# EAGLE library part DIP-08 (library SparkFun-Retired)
DIP Switch 8 Position
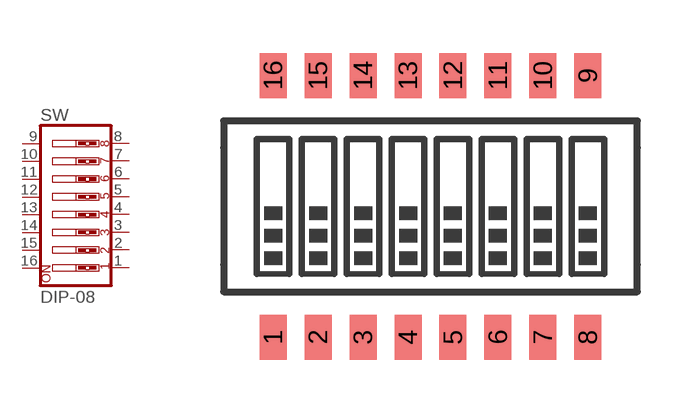
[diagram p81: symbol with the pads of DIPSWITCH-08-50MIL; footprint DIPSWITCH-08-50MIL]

Designator prefix SW

## DIP-08-SMT-HALFSIZE  [DIPSWITCH-08-50MIL]
1  1  pas
2  2  pas
3  3  pas
4  4  pas
5  5  pas
6  6  pas
7  7  pas
8  8  pas
9  9  pas
10  10  pas
11  11  pas
12  12  pas
13  13  pas
14  14  pas
15  15  pas
16  16  pas

## Footprint DIPSWITCH-08-50MIL (pad centres in mm)
DIP SWITCH Half-size SMT DIP switch, 1.27 mm / 0.05" pitch. For example the following: Omron A6H series; Datasheet
smd 0.762 x 1.27: 1 -4.445,-3.7; 2 -3.175,-3.7; 3 -1.905,-3.7; 4 -0.635,-3.7; 5 0.635,-3.7; 6 1.905,-3.7; 7 3.175,-3.7; 8 4.445,-3.7; 9 4.445,3.7; 10 3.175,3.7; 11 1.905,3.7; 12 0.635,3.7; 13 -0.635,3.7; 14 -1.905,3.7; 15 -3.175,3.7; 16 -4.445,3.7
